(* Logix 5000 AddOnInstructionDefinition export Banner_Q90R_KD_Param_v4; software revision 33.00; part 3 of 3 *)
(* tags used below, declared in another part *)
   Q90RKD : Banner_Q90RKD_v4;
   Port_Data : Banner_IOL_Port_v4;
   Port : DINT;
   Local_Control : DINT;
   Command_Being_Processed : BOOL;
   Update_Archive : BOOL;
   Index_Write_Inprocess : DINT;
   Inprocess_Index : DINT;
(* Banner_Q90R_KD_Param_v4, continued *)

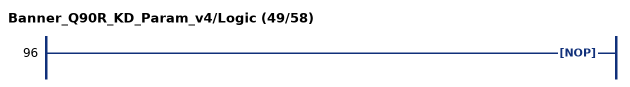
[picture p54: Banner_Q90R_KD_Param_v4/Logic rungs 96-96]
   96: NOP();
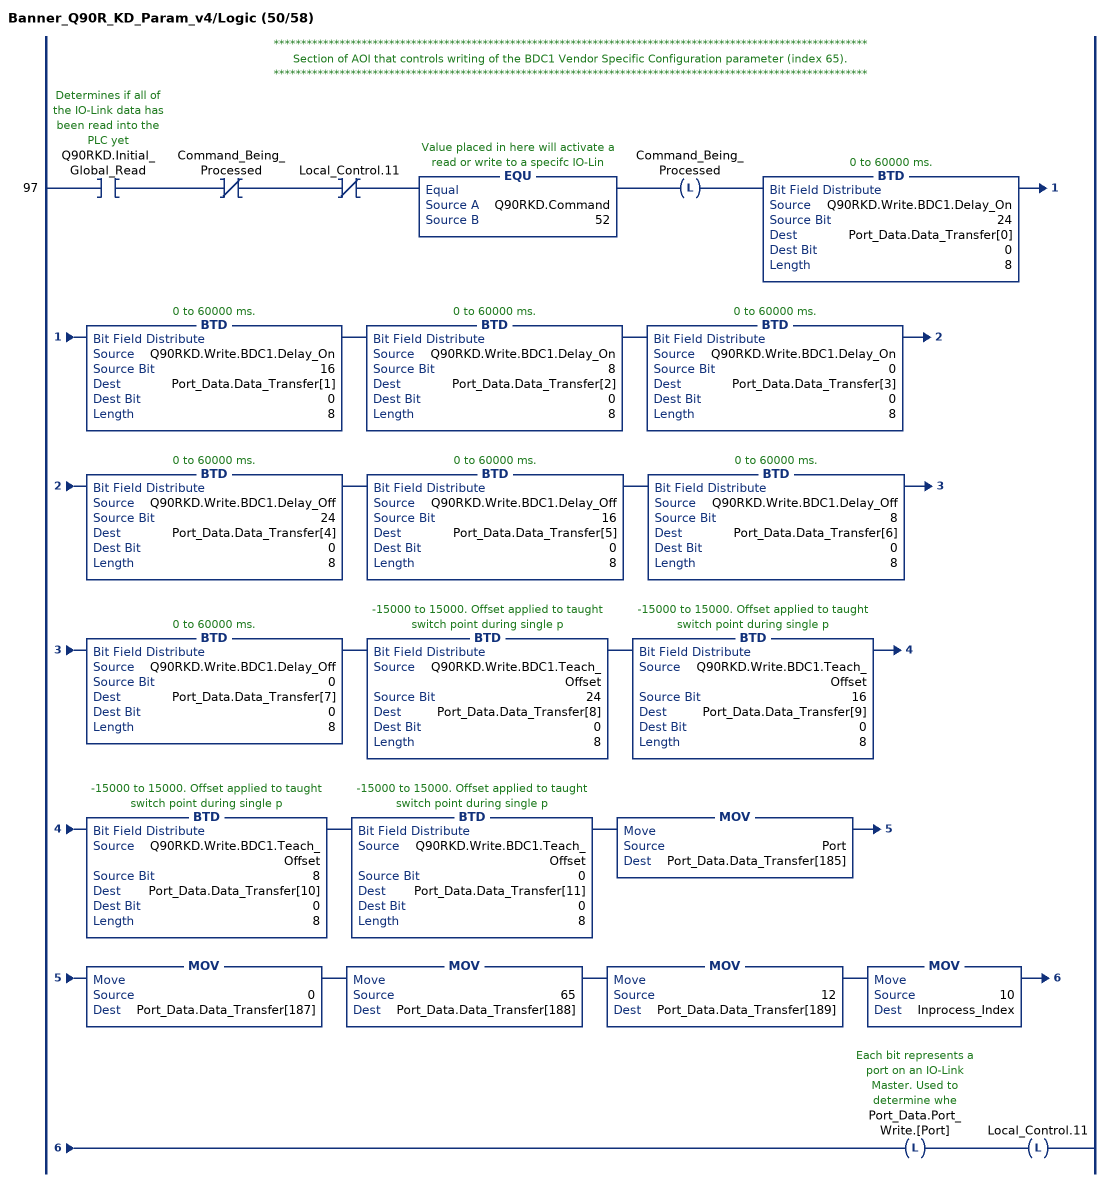
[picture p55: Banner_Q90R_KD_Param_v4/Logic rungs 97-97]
   // ************************************************************************************************************
   // Section of AOI that controls writing of the BDC1 Vendor Specific Configuration parameter (index 65).
   // ************************************************************************************************************
   97: XIC(Q90RKD.Initial_Global_Read)XIO(Command_Being_Processed)XIO(Local_Control.11)EQU(Q90RKD.Command,52)OTL(Command_Being_Processed)BTD(Q90RKD.Write.BDC1.Delay_On,24,Port_Data.Data_Transfer[0],0,8)BTD(Q90RKD.Write.BDC1.Delay_On,16,Port_Data.Data_Transfer[1],0,8)BTD(Q90RKD.Write.BDC1.Delay_On,8,Port_Data.Data_Transfer[2],0,8)BTD(Q90RKD.Write.BDC1.Delay_On,0,Port_Data.Data_Transfer[3],0,8)BTD(Q90RKD.Write.BDC1.Delay_Off,24,Port_Data.Data_Transfer[4],0,8)BTD(Q90RKD.Write.BDC1.Delay_Off,16,Port_Data.Data_Transfer[5],0,8)BTD(Q90RKD.Write.BDC1.Delay_Off,8,Port_Data.Data_Transfer[6],0,8)BTD(Q90RKD.Write.BDC1.Delay_Off,0,Port_Data.Data_Transfer[7],0,8)BTD(Q90RKD.Write.BDC1.Teach_Offset,24,Port_Data.Data_Transfer[8],0,8)BTD(Q90RKD.Write.BDC1.Teach_Offset,16,Port_Data.Data_Transfer[9],0,8)BTD(Q90RKD.Write.BDC1.Teach_Offset,8,Port_Data.Data_Transfer[10],0,8)BTD(Q90RKD.Write.BDC1.Teach_Offset,0,Port_Data.Data_Transfer[11],0,8)MOV(Port,Port_Data.Data_Transfer[185])MOV(0,Port_Data.Data_Transfer[187])MOV(65,Port_Data.Data_Transfer[188])MOV(12,Port_Data.Data_Transfer[189])MOV(10,Inprocess_Index)OTL(Port_Data.Port_Write.[Port])OTL(Local_Control.11);
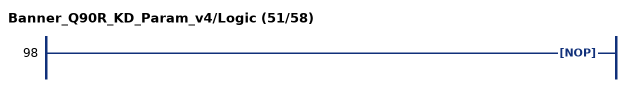
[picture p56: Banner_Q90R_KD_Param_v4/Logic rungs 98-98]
   98: NOP();
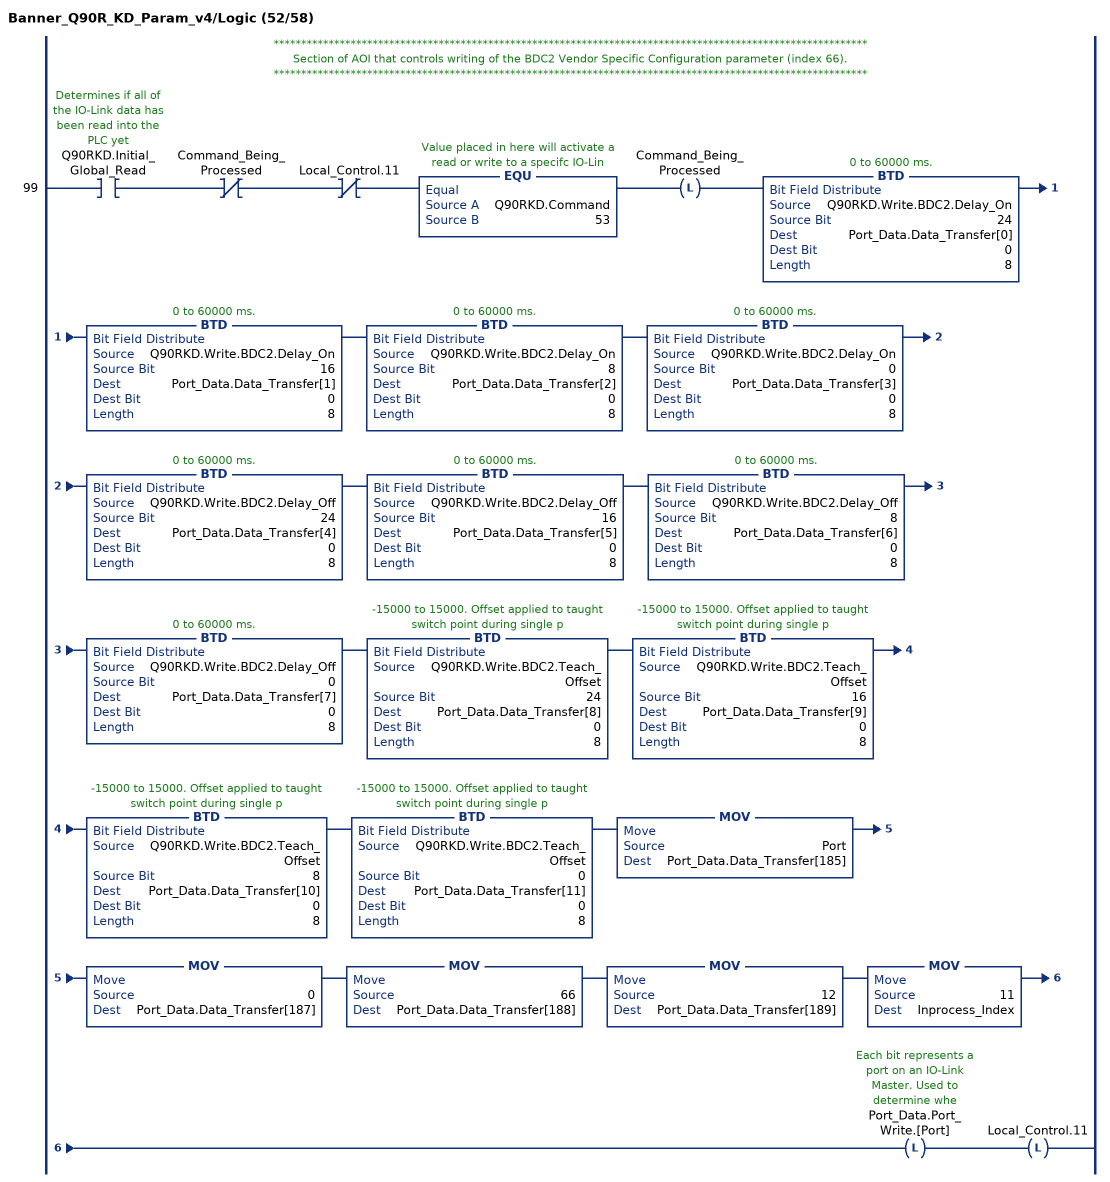
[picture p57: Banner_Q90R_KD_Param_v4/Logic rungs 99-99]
   // ************************************************************************************************************
   // Section of AOI that controls writing of the BDC2 Vendor Specific Configuration parameter (index 66).
   // ************************************************************************************************************
   99: XIC(Q90RKD.Initial_Global_Read)XIO(Command_Being_Processed)XIO(Local_Control.11)EQU(Q90RKD.Command,53)OTL(Command_Being_Processed)BTD(Q90RKD.Write.BDC2.Delay_On,24,Port_Data.Data_Transfer[0],0,8)BTD(Q90RKD.Write.BDC2.Delay_On,16,Port_Data.Data_Transfer[1],0,8)BTD(Q90RKD.Write.BDC2.Delay_On,8,Port_Data.Data_Transfer[2],0,8)BTD(Q90RKD.Write.BDC2.Delay_On,0,Port_Data.Data_Transfer[3],0,8)BTD(Q90RKD.Write.BDC2.Delay_Off,24,Port_Data.Data_Transfer[4],0,8)BTD(Q90RKD.Write.BDC2.Delay_Off,16,Port_Data.Data_Transfer[5],0,8)BTD(Q90RKD.Write.BDC2.Delay_Off,8,Port_Data.Data_Transfer[6],0,8)BTD(Q90RKD.Write.BDC2.Delay_Off,0,Port_Data.Data_Transfer[7],0,8)BTD(Q90RKD.Write.BDC2.Teach_Offset,24,Port_Data.Data_Transfer[8],0,8)BTD(Q90RKD.Write.BDC2.Teach_Offset,16,Port_Data.Data_Transfer[9],0,8)BTD(Q90RKD.Write.BDC2.Teach_Offset,8,Port_Data.Data_Transfer[10],0,8)BTD(Q90RKD.Write.BDC2.Teach_Offset,0,Port_Data.Data_Transfer[11],0,8)MOV(Port,Port_Data.Data_Transfer[185])MOV(0,Port_Data.Data_Transfer[187])MOV(66,Port_Data.Data_Transfer[188])MOV(12,Port_Data.Data_Transfer[189])MOV(11,Inprocess_Index)OTL(Port_Data.Port_Write.[Port])OTL(Local_Control.11);
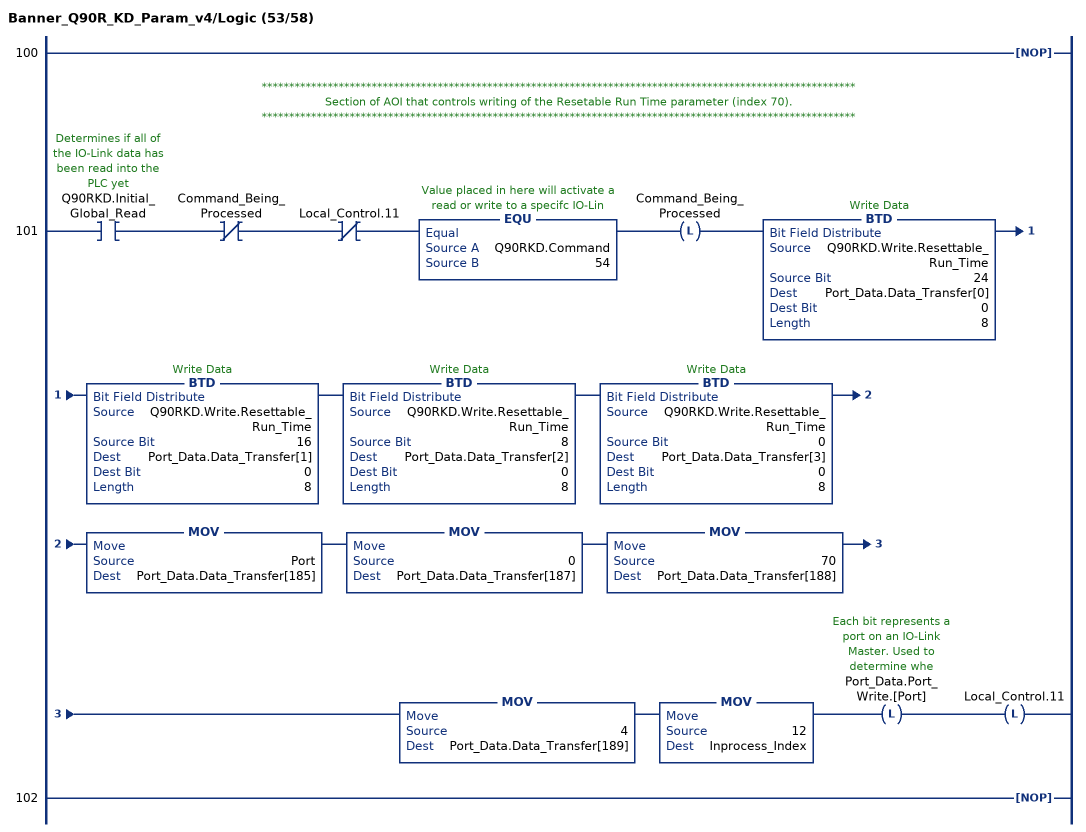
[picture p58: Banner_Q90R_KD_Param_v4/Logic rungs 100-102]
   100: NOP();
   // ************************************************************************************************************
   // Section of AOI that controls writing of the Resetable Run Time parameter (index 70).
   // ************************************************************************************************************
   101: XIC(Q90RKD.Initial_Global_Read)XIO(Command_Being_Processed)XIO(Local_Control.11)EQU(Q90RKD.Command,54)OTL(Command_Being_Processed)BTD(Q90RKD.Write.Resettable_Run_Time,24,Port_Data.Data_Transfer[0],0,8)BTD(Q90RKD.Write.Resettable_Run_Time,16,Port_Data.Data_Transfer[1],0,8)BTD(Q90RKD.Write.Resettable_Run_Time,8,Port_Data.Data_Transfer[2],0,8)BTD(Q90RKD.Write.Resettable_Run_Time,0,Port_Data.Data_Transfer[3],0,8)MOV(Port,Port_Data.Data_Transfer[185])MOV(0,Port_Data.Data_Transfer[187])MOV(70,Port_Data.Data_Transfer[188])MOV(4,Port_Data.Data_Transfer[189])MOV(12,Inprocess_Index)OTL(Port_Data.Port_Write.[Port])OTL(Local_Control.11);
   102: NOP();
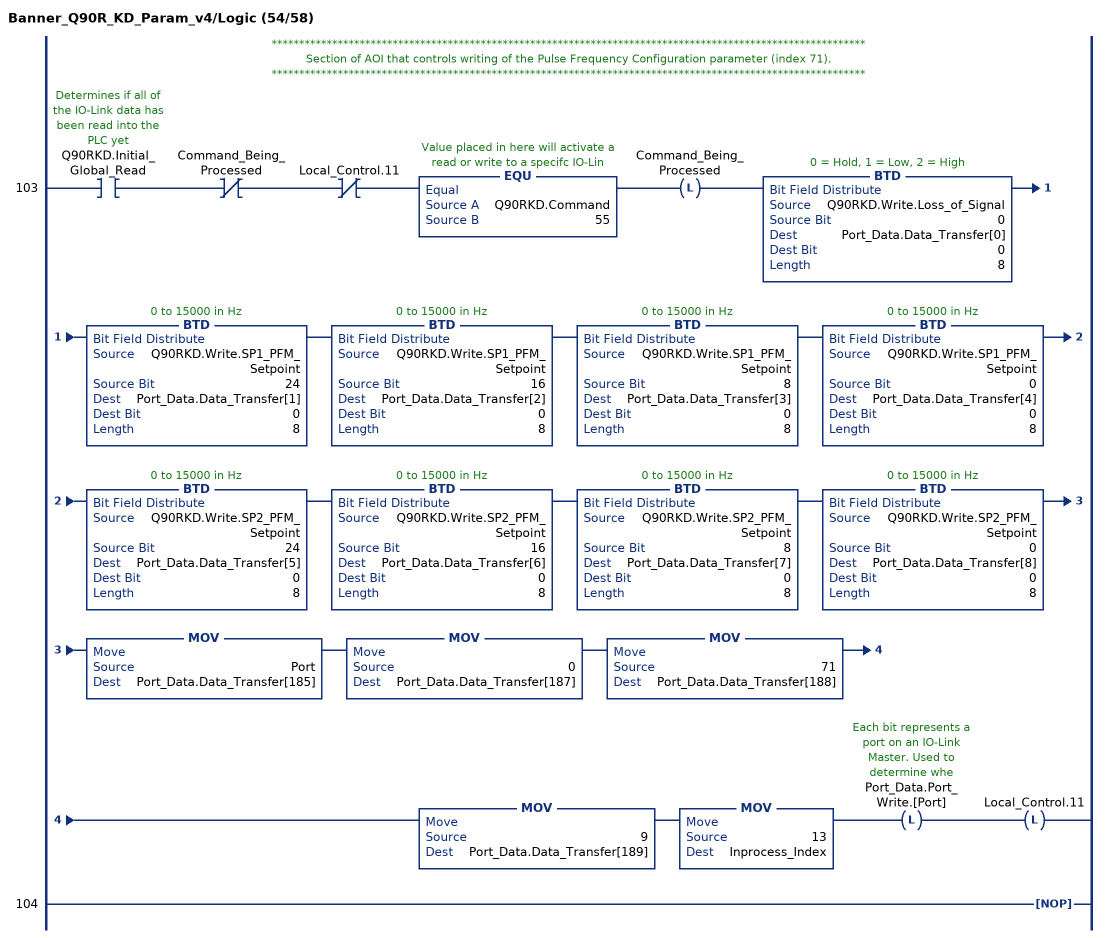
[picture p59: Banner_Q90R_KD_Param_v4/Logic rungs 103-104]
   // ************************************************************************************************************
   // Section of AOI that controls writing of the Pulse Frequency Configuration parameter (index 71).
   // ************************************************************************************************************
   103: XIC(Q90RKD.Initial_Global_Read)XIO(Command_Being_Processed)XIO(Local_Control.11)EQU(Q90RKD.Command,55)OTL(Command_Being_Processed)BTD(Q90RKD.Write.Loss_of_Signal,0,Port_Data.Data_Transfer[0],0,8)BTD(Q90RKD.Write.SP1_PFM_Setpoint,24,Port_Data.Data_Transfer[1],0,8)BTD(Q90RKD.Write.SP1_PFM_Setpoint,16,Port_Data.Data_Transfer[2],0,8)BTD(Q90RKD.Write.SP1_PFM_Setpoint,8,Port_Data.Data_Transfer[3],0,8)BTD(Q90RKD.Write.SP1_PFM_Setpoint,0,Port_Data.Data_Transfer[4],0,8)BTD(Q90RKD.Write.SP2_PFM_Setpoint,24,Port_Data.Data_Transfer[5],0,8)BTD(Q90RKD.Write.SP2_PFM_Setpoint,16,Port_Data.Data_Transfer[6],0,8)BTD(Q90RKD.Write.SP2_PFM_Setpoint,8,Port_Data.Data_Transfer[7],0,8)BTD(Q90RKD.Write.SP2_PFM_Setpoint,0,Port_Data.Data_Transfer[8],0,8)MOV(Port,Port_Data.Data_Transfer[185])MOV(0,Port_Data.Data_Transfer[187])MOV(71,Port_Data.Data_Transfer[188])MOV(9,Port_Data.Data_Transfer[189])MOV(13,Inprocess_Index)OTL(Port_Data.Port_Write.[Port])OTL(Local_Control.11);
   104: NOP();
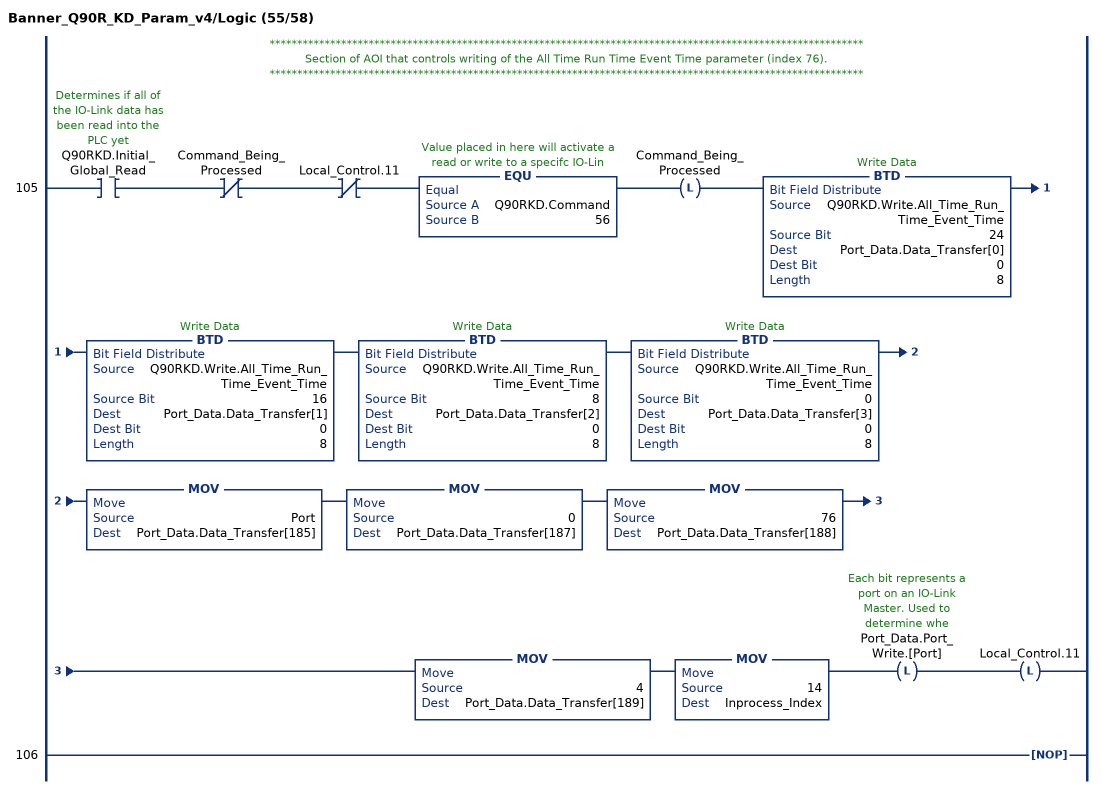
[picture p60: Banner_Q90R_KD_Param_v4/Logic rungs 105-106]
   // ************************************************************************************************************
   // Section of AOI that controls writing of the All Time Run Time Event Time parameter (index 76).
   // ************************************************************************************************************
   105: XIC(Q90RKD.Initial_Global_Read)XIO(Command_Being_Processed)XIO(Local_Control.11)EQU(Q90RKD.Command,56)OTL(Command_Being_Processed)BTD(Q90RKD.Write.All_Time_Run_Time_Event_Time,24,Port_Data.Data_Transfer[0],0,8)BTD(Q90RKD.Write.All_Time_Run_Time_Event_Time,16,Port_Data.Data_Transfer[1],0,8)BTD(Q90RKD.Write.All_Time_Run_Time_Event_Time,8,Port_Data.Data_Transfer[2],0,8)BTD(Q90RKD.Write.All_Time_Run_Time_Event_Time,0,Port_Data.Data_Transfer[3],0,8)MOV(Port,Port_Data.Data_Transfer[185])MOV(0,Port_Data.Data_Transfer[187])MOV(76,Port_Data.Data_Transfer[188])MOV(4,Port_Data.Data_Transfer[189])MOV(14,Inprocess_Index)OTL(Port_Data.Port_Write.[Port])OTL(Local_Control.11);
   106: NOP();
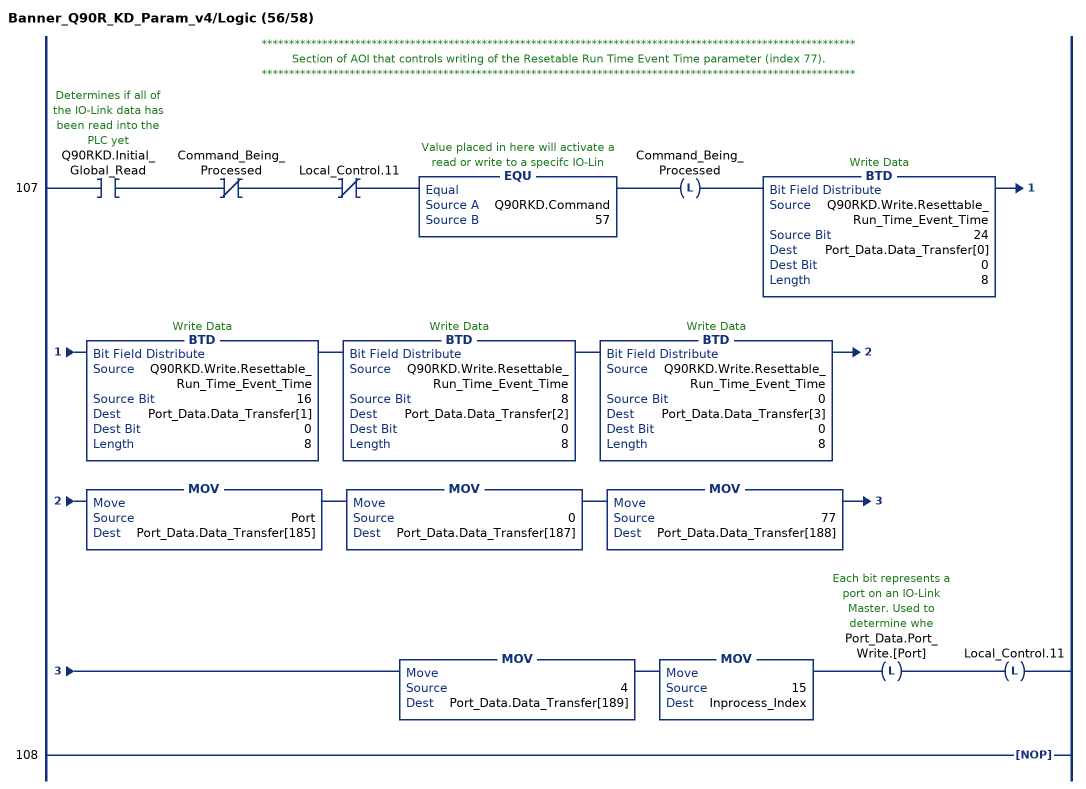
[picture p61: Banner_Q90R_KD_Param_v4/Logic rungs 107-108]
   // ************************************************************************************************************
   // Section of AOI that controls writing of the Resetable Run Time Event Time parameter (index 77).
   // ************************************************************************************************************
   107: XIC(Q90RKD.Initial_Global_Read)XIO(Command_Being_Processed)XIO(Local_Control.11)EQU(Q90RKD.Command,57)OTL(Command_Being_Processed)BTD(Q90RKD.Write.Resettable_Run_Time_Event_Time,24,Port_Data.Data_Transfer[0],0,8)BTD(Q90RKD.Write.Resettable_Run_Time_Event_Time,16,Port_Data.Data_Transfer[1],0,8)BTD(Q90RKD.Write.Resettable_Run_Time_Event_Time,8,Port_Data.Data_Transfer[2],0,8)BTD(Q90RKD.Write.Resettable_Run_Time_Event_Time,0,Port_Data.Data_Transfer[3],0,8)MOV(Port,Port_Data.Data_Transfer[185])MOV(0,Port_Data.Data_Transfer[187])MOV(77,Port_Data.Data_Transfer[188])MOV(4,Port_Data.Data_Transfer[189])MOV(15,Inprocess_Index)OTL(Port_Data.Port_Write.[Port])OTL(Local_Control.11);
   108: NOP();
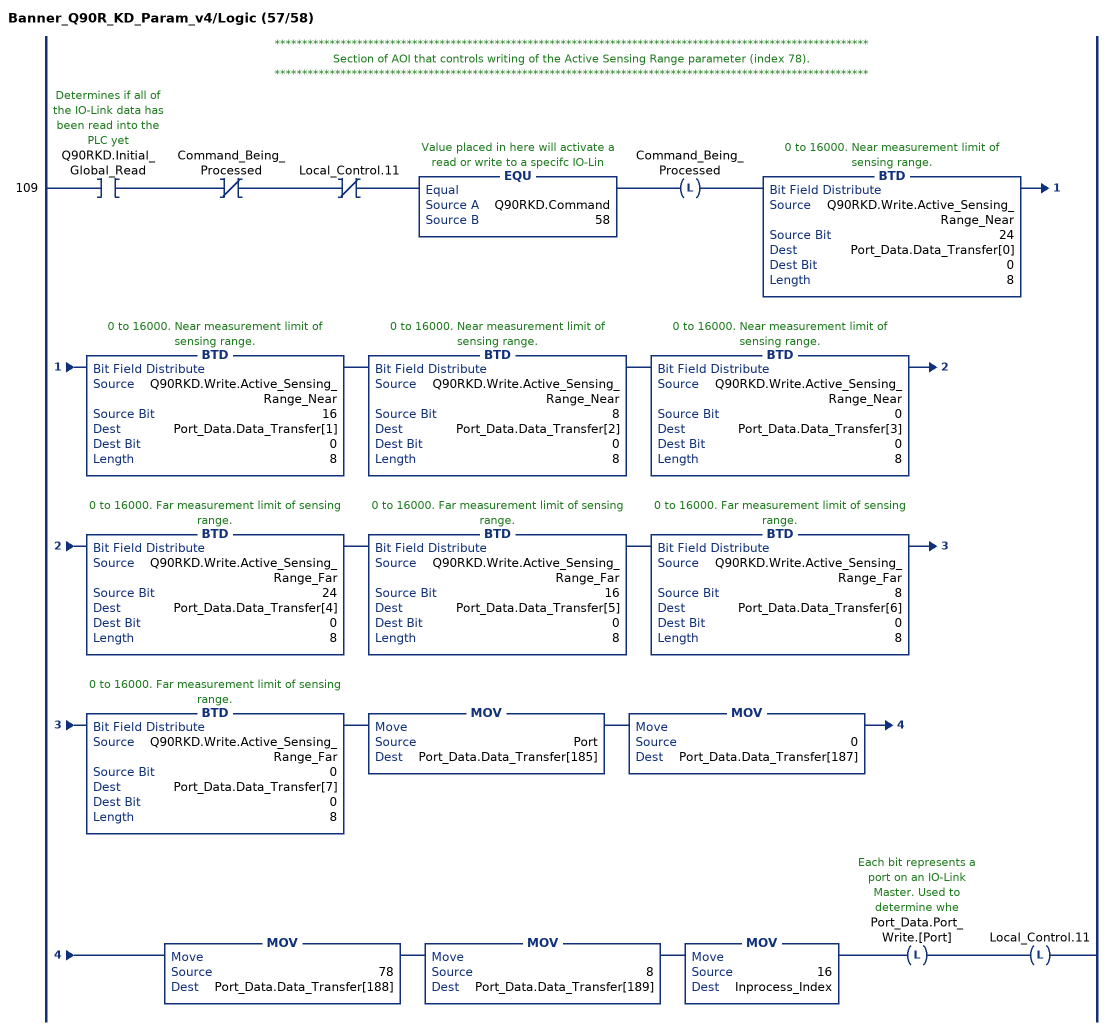
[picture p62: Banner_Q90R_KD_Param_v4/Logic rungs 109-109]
   // ************************************************************************************************************
   // Section of AOI that controls writing of the Active Sensing Range parameter (index 78).
   // ************************************************************************************************************
   109: XIC(Q90RKD.Initial_Global_Read)XIO(Command_Being_Processed)XIO(Local_Control.11)EQU(Q90RKD.Command,58)OTL(Command_Being_Processed)BTD(Q90RKD.Write.Active_Sensing_Range_Near,24,Port_Data.Data_Transfer[0],0,8)BTD(Q90RKD.Write.Active_Sensing_Range_Near,16,Port_Data.Data_Transfer[1],0,8)BTD(Q90RKD.Write.Active_Sensing_Range_Near,8,Port_Data.Data_Transfer[2],0,8)BTD(Q90RKD.Write.Active_Sensing_Range_Near,0,Port_Data.Data_Transfer[3],0,8)BTD(Q90RKD.Write.Active_Sensing_Range_Far,24,Port_Data.Data_Transfer[4],0,8)BTD(Q90RKD.Write.Active_Sensing_Range_Far,16,Port_Data.Data_Transfer[5],0,8)BTD(Q90RKD.Write.Active_Sensing_Range_Far,8,Port_Data.Data_Transfer[6],0,8)BTD(Q90RKD.Write.Active_Sensing_Range_Far,0,Port_Data.Data_Transfer[7],0,8)MOV(Port,Port_Data.Data_Transfer[185])MOV(0,Port_Data.Data_Transfer[187])MOV(78,Port_Data.Data_Transfer[188])MOV(8,Port_Data.Data_Transfer[189])MOV(16,Inprocess_Index)OTL(Port_Data.Port_Write.[Port])OTL(Local_Control.11);
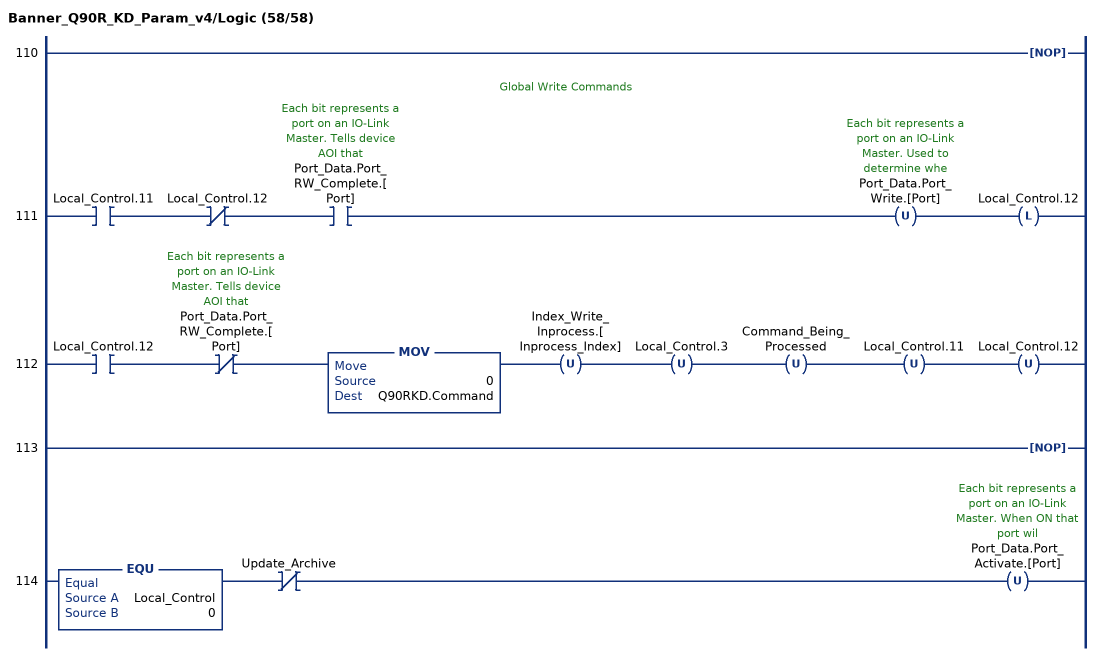
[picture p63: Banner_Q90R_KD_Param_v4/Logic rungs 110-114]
   110: NOP();
   // Global Write Commands
   111: XIC(Local_Control.11)XIO(Local_Control.12)XIC(Port_Data.Port_RW_Complete.[Port])OTU(Port_Data.Port_Write.[Port])OTL(Local_Control.12);
   112: XIC(Local_Control.12)XIO(Port_Data.Port_RW_Complete.[Port])MOV(0,Q90RKD.Command)OTU(Index_Write_Inprocess.[Inprocess_Index])OTU(Local_Control.3)OTU(Command_Being_Processed)OTU(Local_Control.11)OTU(Local_Control.12);
   113: NOP();
   114: EQU(Local_Control,0)XIO(Update_Archive)OTU(Port_Data.Port_Activate.[Port]);
END_ROUTINE
END_ADD_ON_INSTRUCTION
